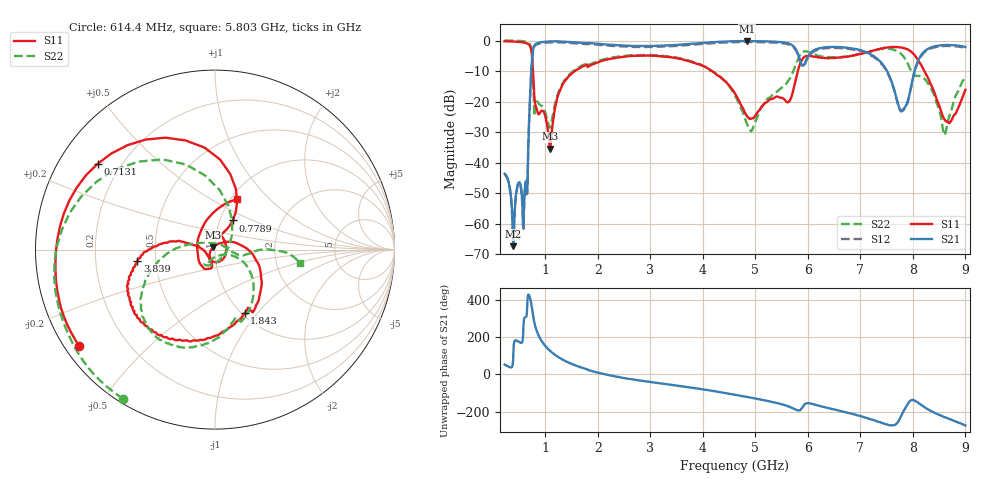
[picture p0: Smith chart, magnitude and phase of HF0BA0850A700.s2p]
!Agilent Technologies,E8358A,US41080443,A.07.50.56
!Agilent E8358A: A.07.50.56
!Date: Friday, July 08, 2016 13:45:57
!Correction: S11(Full 2 Port(1,2))
!S21(Full 2 Port(1,2))
!S12(Full 2 Port(1,2))
!S22(Full 2 Port(1,2))
!S2P File: Measurements: S11, S21, S12, S22:
# Hz S  dB  R 50
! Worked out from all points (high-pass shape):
!   1601 points, 225 MHz to 9 GHz, reference 50 ohm
!   highest |S21| = -0.03 dB at 4.843 GHz (marker M1); lowest = -67.4 dB at 389.5 MHz (marker M2)
!   |S21| within 3 dB of the highest: 765.5 MHz to 5.78 GHz (5.015 GHz wide, 153 % of centre); 6.129 GHz to 7.006 GHz (876.9 MHz wide, 13.4 % of centre)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
!   lowest |S11| = -35.4 dB at 1.092 GHz (marker M3), VSWR 1.03, Z = 48.8 + j1.14 ohm
!   |S11| at or under -10 dB: 765.9 MHz to 1.556 GHz (789.7 MHz wide, 68 % of centre); 4.183 GHz to 5.807 GHz (1.624 GHz wide, 32.5 % of centre); 8.222 GHz to end of sweep
!   |S22| runs from -31.0 to 0.1 dB; largest |S21 - S12| = 0.039
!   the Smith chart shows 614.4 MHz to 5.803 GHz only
!   S11 on the Smith chart (normalised r, x): 614.4 MHz: 0.04, -0.32; 713.1 MHz: 0.12, +0.32; 778.9 MHz: 1.15, +0.39; 1.843 GHz: 1.03, -0.86; 3.839 GHz: 0.39, -0.06; 5.803 GHz: 1.07, +0.66
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2.25e8  -0.12 -40.5  -43.62 52.3  -43.95 53.0  0.14 -34.3
3.895312e8  -0.20 -74.1  -67.42 89.8  -67.15 91.6  0.09 -62.6
6.143906e8  -0.64 -144.8  -47.69 -54.6  -48.05 -54.3  -0.21 -121.7
7.131094e8  -1.83 143.8  -16.83 45.3  -17.16 45.5  -1.31 172.6
7.789219e8  -14.42 58.6  -2.00 -64.7  -2.33 -64.5  -17.65 43.0
9.050625e8  -23.37 -42.7  -0.48 -169.5  -0.83 -169.4  -21.03 -121.3
1.091531e9  -35.44 136.2  -0.16 125.6  -0.50 125.8  -28.38 -63.5
1.288969e9  -15.88 6.0  -0.18 85.3  -0.52 85.5  -15.27 -23.7
1.689328e9  -8.55 -49.4  -0.64 36.1  -0.97 36.3  -8.18 -61.1
1.842891e9  -8.19 -64.9  -0.69 20.8  -1.02 20.9  -7.74 -75.5
3.153656e9  -5.03 -144.9  -1.61 -47.3  -1.95 -47.1  -4.78 -128.9
3.839203e9  -7.19 -171.6  -0.88 -73.9  -1.19 -73.8  -7.03 -153.1
4.6125e9  -17.31 167.4  -0.11 -109.9  -0.42 -109.8  -17.93 164.7
4.842844e9  -24.80 -171.1  -0.03 -121.8  -0.37 -121.8  -27.45 119.2
5.802609e9  -10.26 66.0  -3.87 166.6  -4.24 166.8  -6.40 -8.7
6.076828e9  -5.04 -42.0  -3.61 -158.3  -3.92 -158.4  -4.13 -71.1
7.042078e9  -4.16 -125.5  -3.29 132.2  -3.58 132.1  -4.03 -157.4
7.541156e9  -2.16 -179.4  -11.10 87.4  -11.40 87.6  -2.57 133.2
7.875703e9  -2.64 128.8  -21.04 -171.7  -21.30 -172.2  -6.53 30.6
8.155406e9  -7.85 73.0  -4.72 -164.2  -5.06 -164.2  -11.57 -159.6
8.605125e9  -25.85 44.0  -1.37 129.9  -1.70 129.8  -30.95 -176.2
9e9  -16.05 12.6  -2.02 85.5  -2.36 85.2  -11.93 -83.9
